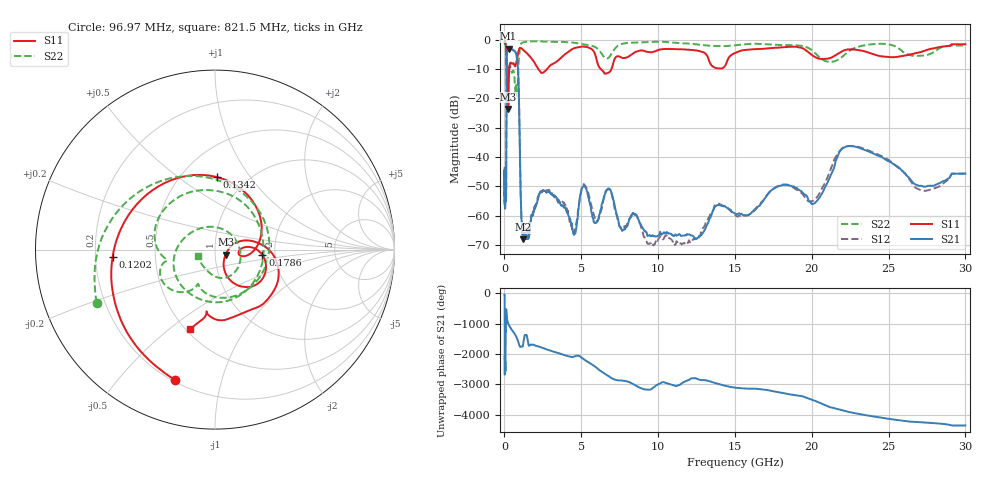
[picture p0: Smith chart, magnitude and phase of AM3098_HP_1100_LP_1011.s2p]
! Date/Time: Thu, Feb 28, 2019 8:44 AM
! Network Analyzer: Agilent Technologies E8364B Rev: A.07.50.67
! Sweep from 0.010 to 30.000 GHz, 1601 Points, Sweep Type: LOG
! Power Supply: 5.022 V, 0.002 A
# Hz S DB R 50
!freq MagS11 AngS11 MagS21 AngS21 MagS12 AngS12 MagS22 AngS22
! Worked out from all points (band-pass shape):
!   1601 points, 10 MHz to 30 GHz, reference 50 ohm
!   highest |S21| = -3.08 dB at 263.8 MHz (marker M1); lowest = -68.1 dB at 1.238 GHz (marker M2)
!   |S21| within 3 dB of the highest: 149.3 MHz to 805.6 MHz (656.3 MHz wide, 137 % of centre)
!   lowest |S11| = -23.6 dB at 247.2 MHz (marker M3), VSWR 1.14, Z = 56.2 - j3.23 ohm
!   |S11| at or under -10 dB: 140.1 MHz to 312.7 MHz (172.6 MHz wide, 76.2 % of centre); 2.193 GHz to 2.78 GHz (586.3 MHz wide, 23.6 % of centre); 6.261 GHz to 6.969 GHz (707.8 MHz wide, 10.7 % of centre)
!   |S22| runs from -20.0 to -0.6 dB; largest |S21 - S12| = 0.012
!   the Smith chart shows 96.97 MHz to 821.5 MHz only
!   S11 on the Smith chart (normalised r, x): 96.97 MHz: 0.21, -0.72; 120.2 MHz: 0.27, -0.03; 134.2 MHz: 0.73, +0.71; 178.6 MHz: 1.71, -0.11; 821.5 MHz: 0.53, -0.60
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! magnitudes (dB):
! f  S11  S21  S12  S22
! 10 MHz  -0.4  -44.6  -44.7  -0.6
! 38.04 MHz  -0.4  -56.2  -55.9  -0.9
! 96.97 MHz  -2.4  -54.0  -52.3  -2.8
! 120.2 MHz  -4.9  -37.0  -37.2  -6.3
! 134.2 MHz  -7.9  -15.5  -15.4  -10.4
! 144.7 MHz  -12.3  -7.5  -7.4  -11.8
! 178.6 MHz  -11.5  -4.0  -4.0  -10.3
! 247.2 MHz  -23.6  -3.1  -3.1  -11.3
! 263.8 MHz  -18.8  -3.1  -3.0  -11.1
! 550.5 MHz  -8.1  -3.6  -3.6  -10.7
! 821.5 MHz  -6.7  -6.6  -6.6  -19.8
! 926.3 MHz  -3.8  -15.8  -15.8  -7.3
! 1.098 GHz  -3.0  -60.6  -60.2  -1.4
! 1.238 GHz  -3.6  -68.1  -68.0  -1.0
! 2.084 GHz  -9.0  -56.1  -56.1  -0.6
! 4.525 GHz  -3.0  -66.6  -65.8  -1.1
! 6.753 GHz  -11.4  -50.7  -51.1  -6.3
! 7.926 GHz  -6.2  -63.9  -63.6  -1.2
! 12.13 GHz  -3.5  -66.7  -68.7  -1.4
! 20.2 GHz  -5.9  -55.7  -54.5  -4.5
! 22.67 GHz  -3.4  -36.4  -36.3  -3.2
! 30 GHz  -1.6  -45.7  -45.7  -2.0
